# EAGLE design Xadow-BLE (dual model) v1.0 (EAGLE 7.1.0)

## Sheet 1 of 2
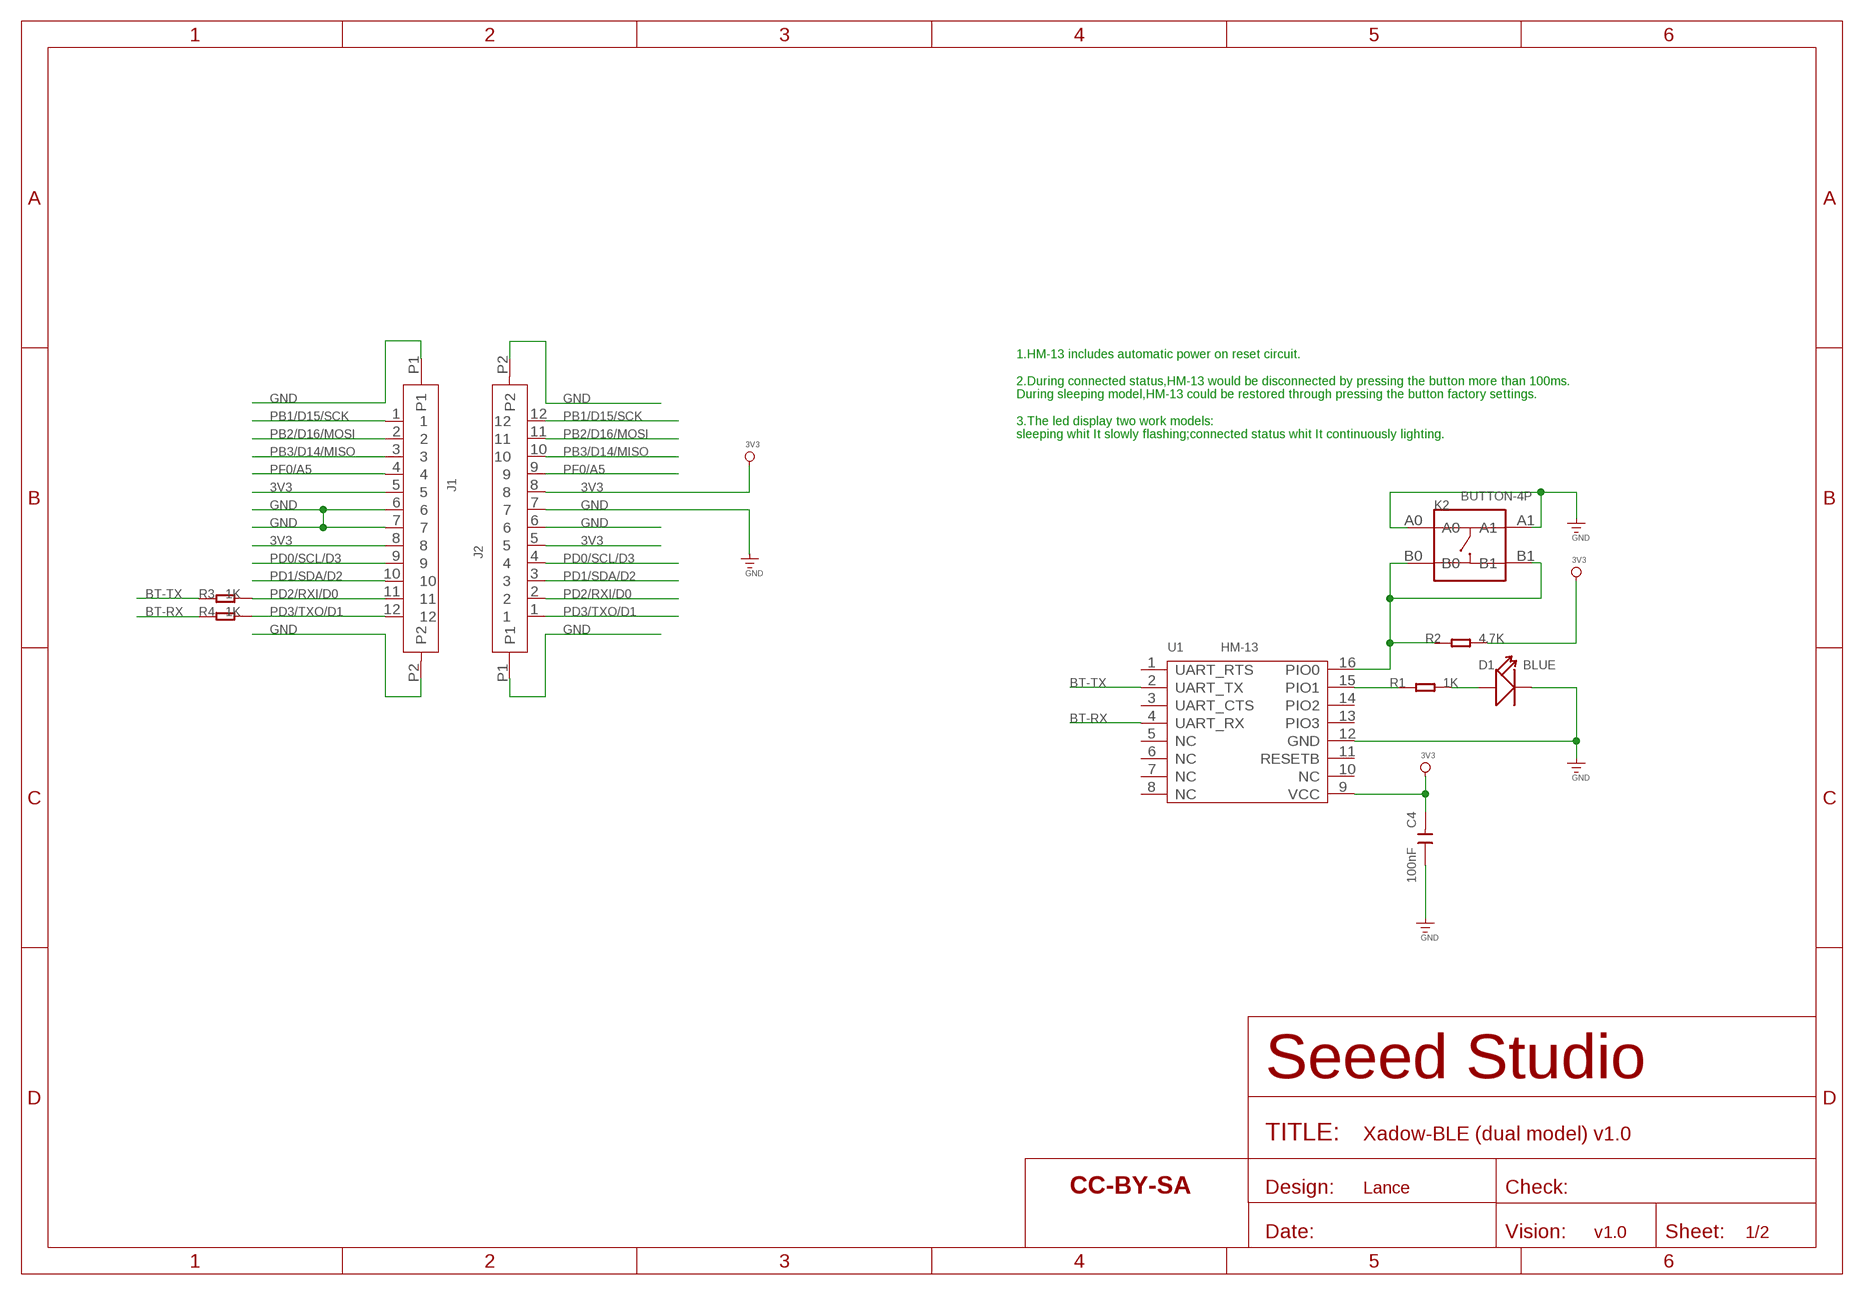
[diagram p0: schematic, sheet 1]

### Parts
C4  100nF  C-0402  [C0402]
D1  BLUE  LED'0603'  [LED-0603]
J1  FPC052002-12LT-FH12-12S-0.5SH  [12P-0.5-NEW]
J2  FPC052002-12LT-FH12-12S-0.5SH  [12P-0.5-NEW]
K2  BUTTON-4P  BUTTON-4P-3.3X3.3  [4P-SMD-L3.35*W3.35*H1.5MM]
R1  1K  R-0402  [R0402]
R2  4.7K  R-0402  [R0402]
R3  1K  R-0402  [R0402]
R4  1K  R-0402  [R0402]
U1  HM-13  MOUDLE-BLUETOOTH-HM-13  [16P-L18.5*W13.5*H2.3MM]
U$1  SEEEDSTUDIO-OPEN-SCH-FRAME  [SEEEDSTUDIO-PCB-FRAME]

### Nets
3V3: C4.2 J1.5 J1.8 J2.5 J2.8 R2.2 U1.9(VCC)
BT-RX: R4.1 U1.4(UART_RX)
BT-TX: R3.1 U1.2(UART_TX)
GND: C4.1 D1.- J1.6 J1.7 J1.P1 J1.P2 J2.6 J2.7 J2.P1 J2.P2 K2.A0 K2.A1 U1.12(GND)
N$7: R1.1 U1.15(PIO1)
N$8: D1.+ R1.2
N$11: K2.B0 K2.B1 R2.1 U1.16(PIO0)
PB1/D15/SCK: J1.1 J2.12
PB2/D16/MOSI: J1.2 J2.11
PB3/D14/MISO: J1.3 J2.10
PD0/SCL/D3: J1.9 J2.4
PD1/SDA/D2: J1.10 J2.3
PD2/RXI/D0: J1.11 J2.2 R3.2
PD3/TXO/D1: J1.12 J2.1 R4.2
PF0/A5: J1.4 J2.9
Unconnected: U1.1(UART_RTS) U1.3(UART_CTS) U1.5(NC) U1.6(NC) U1.7(NC) U1.8(NC) U1.10(NC) U1.11(RESETB) U1.13(PIO3) U1.14(PIO2)

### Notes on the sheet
- 1.HM-13 includes automatic power on reset circuit.
   
  2.During connected status,HM-13 would be disconnected by pressing the button more than 100ms.
  During sleeping model,HM-13 could be restored through pressing the button factory settings.
  
  3.The led display two work models:
  sleeping whit It slowly flashing;connected status whit It continuously lighting.
- Lance
- v1.0

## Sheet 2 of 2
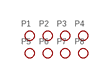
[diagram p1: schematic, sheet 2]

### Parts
P1  PAD-MARK  [ROUND-MARK-1.0]
P2  PAD-MARK  [ROUND-MARK-1.0]
P3  PAD-MARK  [ROUND-MARK-1.0]
P4  PAD-MARK  [ROUND-MARK-1.0]
P5  PAD-MARK  [ROUND-MARK-1.0]
P6  PAD-MARK  [ROUND-MARK-1.0]
P7  PAD-MARK  [ROUND-MARK-1.0]
P8  PAD-MARK  [ROUND-MARK-1.0]

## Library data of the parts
C4 = Discrete:C*: Ceramic Capacitors
D1 = Discrete-new:LED
J1 J2 = template:FPC052002-12LT
K2 = Discrete-new:BUTTON-4P: 4P-L6.0*W6.0*H5.0mm:311020024;4P-L8.0*W8.0*H9.0MM:311020028;4P-SMD-L6.0*W6.0*H5.0MM:311020004;4P-SMD-L3.35*W3.35*H1.5MM:311020030;4P-SMD-L5.2*W5.2*H2.5:311020046
P1-P8 = Discrete:PAD-MARK; PARTNO: DNP
R1-R4 = Discrete:R*
U1 = template:MOUDLE-BLUETOOTH-HM-13: Bluetooth Specification V4.0 EDR and BLE
U$1 = moudle-new:SEEEDSTUDIO-OPEN-SCH-FRAME

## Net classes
0 default: width 0.152 mm, drill 0.305 mm, clearance 0.152 mm
1 GND: width 0.152 mm, drill 0.305 mm, clearance 0.152 mm to class 0, clearance 0.152 mm

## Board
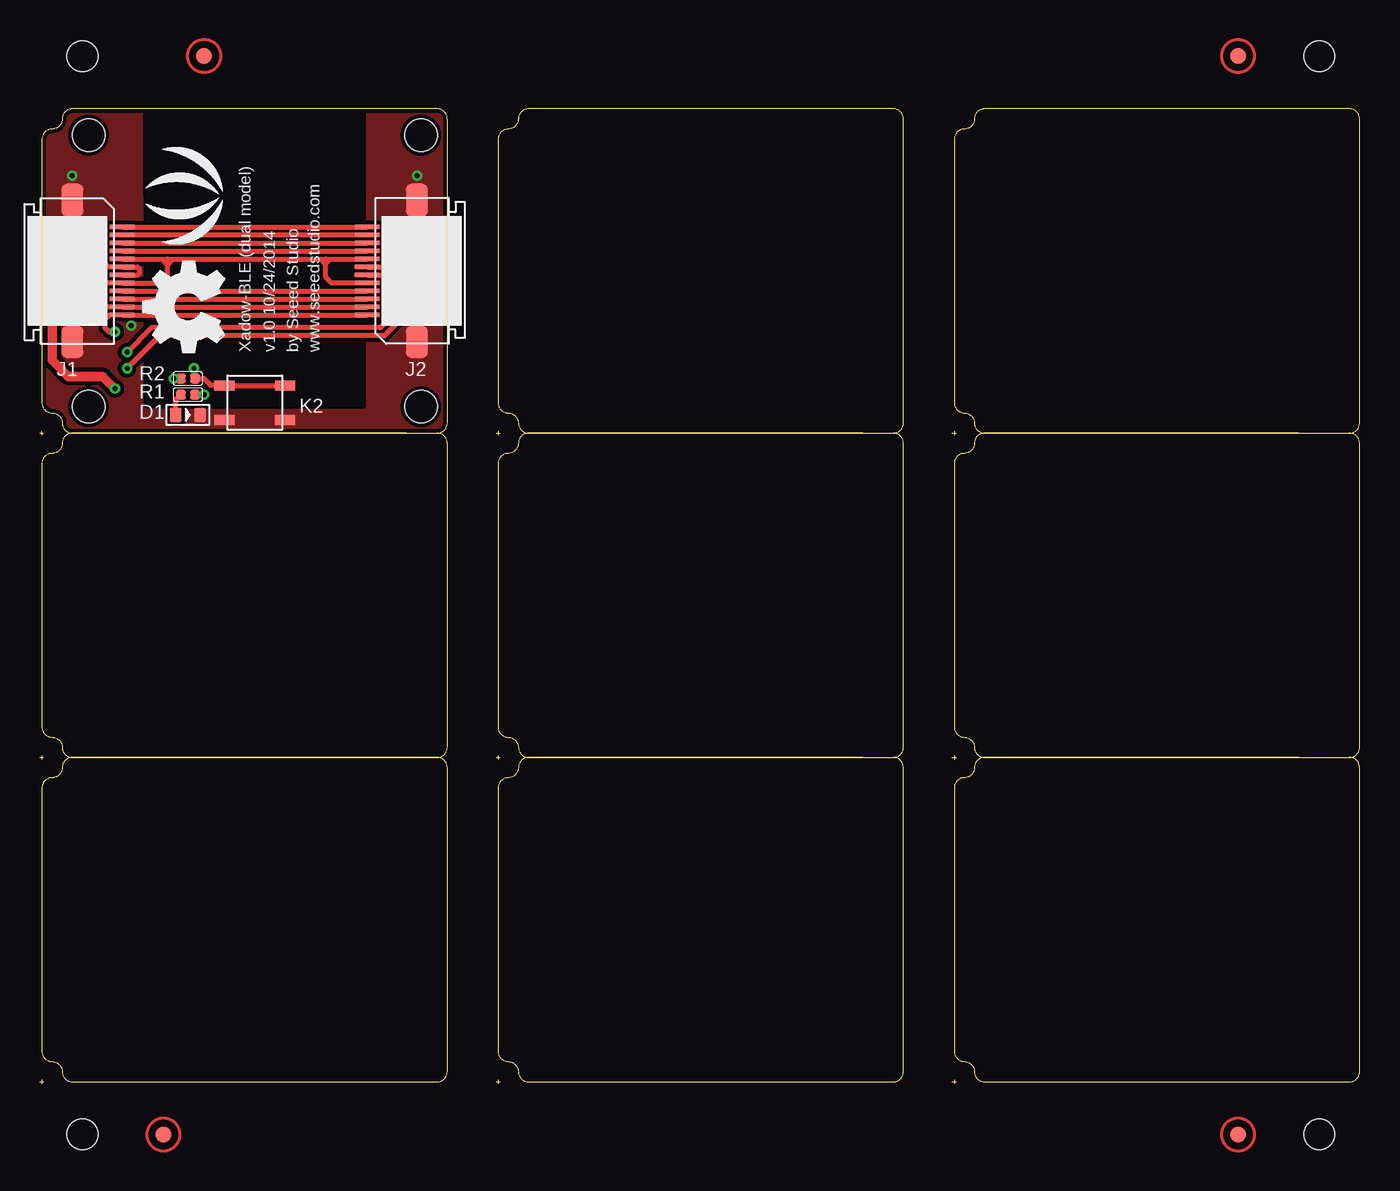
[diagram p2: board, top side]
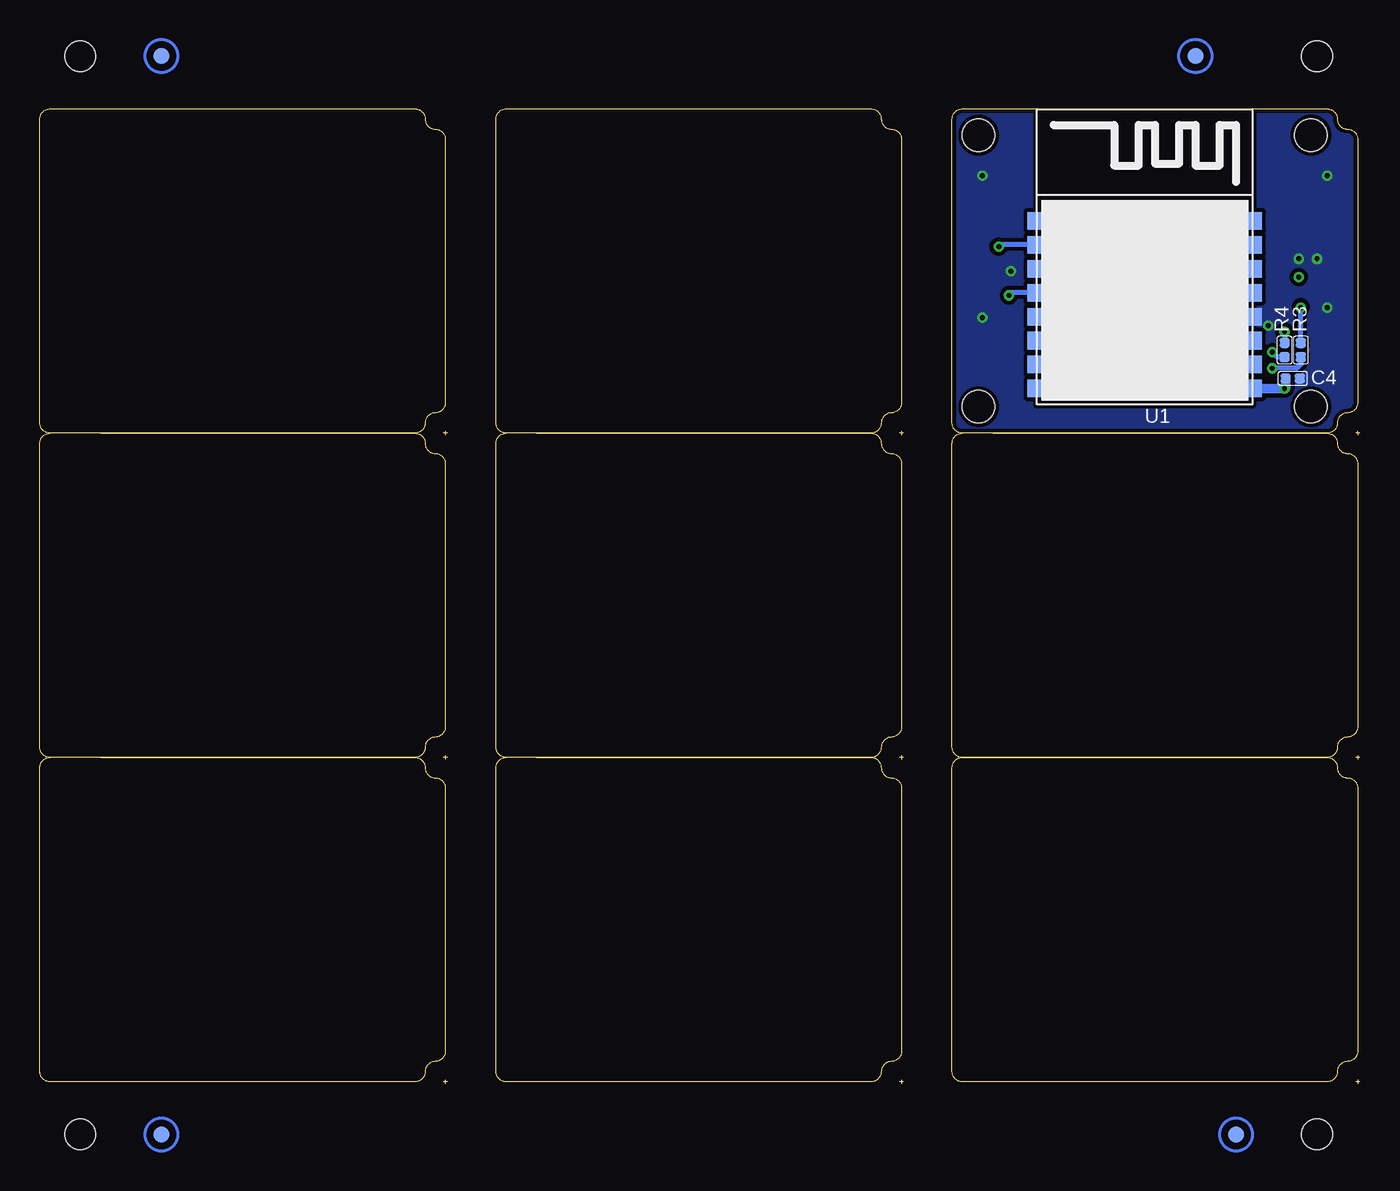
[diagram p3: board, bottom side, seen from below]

Size 82.68 x 61.09 mm. Coordinates in mm from the lower left corner, seen from the top.
Outline: 217 segments
Copper layers (1*16): Top 0.035mm / dielectric 1.5mm / Bottom 0.035mm
Design rules "SeeedStudio_2layer_DRU_no_angle_20140221 *": minimum track width 6mil, minimum drill 12mil, track to track 6mil, track to pad 6mil, pad to pad 6mil, via to via 6mil, smd to smd 0mil, copper to edge 10mil, drill to drill 10mil, minimum pad ring 10mil, minimum via ring 6mil, stop-mask expansion 2mil, vias tented up to drill 100mil, thermal gap 10mil
Holes 2.03 mm at 3.05,42.42 3.05,59.44 23.88,59.44 23.88,42.42
Holes 1.91 mm at 80.14,64.39 2.67,64.39 2.67,-3.17 80.14,-3.17
tRestrict: area 6.7,42.5 to 20.2,61.1; 21 lines
bRestrict: area 6.7,42.5 to 20.2,61.1; 21 lines

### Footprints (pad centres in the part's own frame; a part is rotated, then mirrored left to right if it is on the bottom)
C0402 = smd 0.635 x 0.635: 1 -0.445,0; 2 0.445,0
LED-0603 = smd 0.762 x 0.889: + -0.762,0; - 0.762,0
12P-0.5-NEW = smd 0.3 x 1.6: 1 -2.75,3.127; 2 -2.25,3.127; 3 -1.75,3.127; 4 -1.25,3.127; 5 -0.75,3.127; 6 -0.25,3.127; 7 0.25,3.127; 8 0.75,3.127; 9 1.25,3.127; 10 1.75,3.127; 11 2.25,3.127; 12 2.75,3.127 | smd 2.032 x 1.397: P1 -4.445,0; P2 4.445,0
4P-SMD-L3.35*W3.35*H1.5MM = smd 1.27 x 0.635: A0 -1.905,1.079; A1 1.905,1.079; B0 -1.905,-1.079; B1 1.905,-1.079
ROUND-MARK-1.0 = smd 1.016 x 1.016: P$1 0,0
R0402 = smd 0.635 x 0.635: 1 -0.445,0; 2 0.445,0
16P-L18.5*W13.5*H2.3MM = smd 1.7 x 1.1: 1 -6.5,2.25; 2 -6.5,0.75; 3 -6.5,-0.75; 4 -6.5,-2.25; 5 -6.5,-3.75; 6 -6.5,-5.25; 7 -6.5,-6.75; 8 -6.5,-8.25; 9 6.5,-8.25; 10 6.5,-6.75; 11 6.5,-5.25; 12 6.5,-3.75; 13 6.5,-2.25; 14 6.5,-0.75; 15 6.5,0.75; 16 6.5,2.25

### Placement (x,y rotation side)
C4  4.19,44.2 180 bottom
D1  9.27,41.91 0 top
J1  2.03,50.93 270 top
J2  23.62,50.93 90 top
K2  13.46,42.67 180 top
P1  not placed on the board
P2  not placed on the board
P3  not placed on the board
P4  not placed on the board
P5  not placed on the board
P6  not placed on the board
P7  not placed on the board
P8  not placed on the board
R1  9.27,43.18 180 top
R2  9.27,44.2 180 top
R3  3.68,45.97 90 bottom
R4  4.7,45.97 90 bottom
U1  13.46,51.82 0 bottom
U$1  not placed on the board
U$2  [LOGO_SILK]  9.78,55.63 90 top
U$3  [OSHW_FILLX200_NOTEXT]  11.56,45.85 90 top

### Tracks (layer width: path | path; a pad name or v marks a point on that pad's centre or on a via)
3V3  (via drill 0.3 pad 0.64)
  Top 0.305: J1.5 8,51.68 | 8,51.68 17.91,51.68 | 17.91,51.68 J2.8 | 19.16,50.18 J2.5 18.28,50.18 17.91,50.55 17.91,51.37 | 8,51.31 8,50.67 7.5,50.18 J1.8 4.18,50.18 v3.81,50.55 | 8,51.31 8,51.68 | 8,51.31 7.68,51.63 | 8,51.31 8.32,51.63 | 17.91,51.37 17.91,51.68 | 17.91,51.37 17.65,51.63 | 17.91,51.37 18.16,51.63
  Top 0.61: v3.81,50.55 1.65,50.55 0.76,49.66 0.76,45.34 1.78,44.32 3.94,44.32 v4.7,43.56 | R2.2 v8.38,44.2
  Bottom 0.61: C4.2 4.64,43.62 v4.7,43.56 v4.7,43.57 U1.9 7.62,43.57 8.25,44.2 v8.38,44.2
BT-RX  (via drill 0.3 pad 0.64)
  Top 0.305: v5.46,45.85 6.99,47.37 21.34,47.37 21.97,48.01 v21.97,49.4
  Bottom 0.305: R4.1 5.14,45.53 v5.46,45.85 | U1.4 21.81,49.57 v21.97,49.4
BT-TX  (via drill 0.3 pad 0.64)
  Top 0.305: v5.46,44.83 7.49,46.86 21.59,46.86 22.73,48.01 22.73,52.32 v22.61,52.45
  Bottom 0.305: R3.1 3.68,45.09 3.94,44.83 v5.46,44.83 | U1.2 22.49,52.57 v22.61,52.45
GND  (via drill 0.3 pad 0.64)
  Top 0.305: 5.08,50.68 J1.7 6.1,50.68 6.22,50.8 6.22,51.05 6.1,51.18 J1.6 4.32,51.18 v3.81,51.69 | J2.7 21.59,51.18 v21.84,50.93 21.59,50.68 J2.6
  other vias: 2.03,48.64 5.71,47.5 2.67,51.69 2.03,56.9 23.62,56.9 23.62,48.01
  pour Top (isolate 0.254, rank 6, no thermals): -0.51,61.72 26.16,61.72 26.16,40.77 -0.51,40.77
  pour Bottom (isolate 0.254, rank 6, no thermals): -0.51,61.72 26.16,61.72 26.16,40.77 -0.51,40.77
N$7  (via drill 0.3 pad 0.64)
  Top 0.305: R1.1 v10.29,43.18
  Bottom 0.305: v10.29,43.18 9.91,43.18 9.02,44.07 9.02,51.69 8.32,52.39 8.25,52.45 8.14,52.57 U1.15
N$8
  Top 0.305: D1.+ 8.51,42.86 R1.2
N$11  (via drill 0.3 pad 0.64)
  Top 0.305: K2.B0 K2.B1 10.73,43.75 10.29,44.2 R2.1 9.72,44.77 v9.65,44.83
  Bottom 0.305: v9.65,44.83 9.65,52.7 8.45,53.91 8.38,53.98 8.29,54.07 U1.16
PB1/D15/SCK
  Top 0.305: J1.1 J2.12
PB2/D16/MOSI
  Top 0.305: J2.11 J1.2
PB3/D14/MISO
  Top 0.305: J1.3 J2.10
PD0/SCL/D3
  Top 0.305: J1.9 J2.4
PD1/SDA/D2
  Top 0.305: J1.10 J2.3
PD2/RXI/D0  (via drill 0.3 pad 0.64)
  Top 0.305: J2.2 J1.11 3.72,48.68 v3.68,48.64
  Bottom 0.305: R3.2 v3.68,48.64
PD3/TXO/D1  (via drill 0.3 pad 0.64)
  Top 0.305: J2.1 J1.12 4.36,48.18 4.06,47.88 4.06,47.37 4.32,47.12 v4.7,47.12
  Bottom 0.305: v4.7,47.12 R4.2
PF0/A5
  Top 0.305: J1.4 J2.9

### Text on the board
tPlace: Xadow-BLE (dual model) | v1.0 10/24/2014 | by Seeed Studio | www.seeedstudio.com
tEnhance: Top Enhance 0.25~0.28mm | Top Enhance 0.25~0.28mm
bEnhance: Bottom Enhance | Bottom Enhance
bEnHoles: Holes on Bottom Enhance | Holes on Bottom Enhance | All Holes are 70mil diameter | All Holes are 70mil diameter

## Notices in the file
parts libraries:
moudle-new: This work is licensed under the Creative Commons Attribution 4.0 International License.
To view a copy of this license,visit:
http://creativecommons.org/licenses/by-sa/4.0
moudle-new: CC-BY-SA
